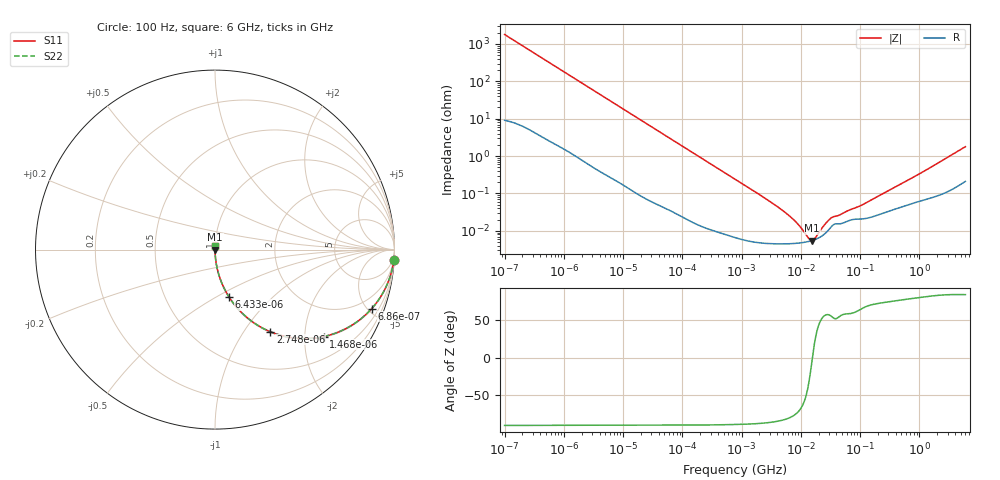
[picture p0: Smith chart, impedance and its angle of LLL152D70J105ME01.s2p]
!Murata Part Number: LLL152D70J105ME01
!These Parameters are Measured in Series Mode Connection
!Data Generated on Jan 08, 2026
!  o--ll--o
!Port1  Port2
!  o------o
!Operation Temp=25[degC], DC Bias Voltage=0[V]
!Freq. Start=100[Hz] Stop=6[GHz] 401[Steps]
# Hz S RI R 50
!Freq.(Hz) S11(Real) S11(Imag) S21(Real) S21(Imag) S12(Real) S12(Imag) S22(Real) S22(Imag)
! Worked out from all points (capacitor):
!   401 points, 100 Hz to 6 GHz, reference 50 ohm
!   read as one part in series: C = 885 nF near 109 Hz
!   lowest |Z| = 5.52 mohm at 15.56 MHz (marker M1)
!   series resonance near 15.7 MHz, so ESL is about 120 pH
!   S11 on the Smith chart (normalised r, x): 100 Hz: 1, -36; 686 Hz: 1.04, -5.29; 1.468 kHz: 1.02, -2.48; 2.748 kHz: 1.01, -1.33; 6.433 kHz: 1.01, -0.57; 6 GHz: 1.00, +0.04
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100  0.9966 -0.0555  0.00337 0.0555  0.00337 0.0555  0.9966 -0.0555
268  0.9774 -0.145  0.0226 0.145  0.0226 0.145  0.9774 -0.145
686  0.8727 -0.3292  0.1273 0.3292  0.1273 0.3292  0.8727 -0.3292
981  0.7721 -0.4153  0.2279 0.4153  0.2279 0.4153  0.7721 -0.4153
1468  0.605 -0.4845  0.395 0.4845  0.395 0.4845  0.605 -0.4845
2008  0.4523 -0.4935  0.5477 0.4935  0.5477 0.4935  0.4523 -0.4935
2748  0.308 -0.4574  0.692 0.4574  0.692 0.4574  0.308 -0.4574
4111  0.1675 -0.3692  0.8325 0.3692  0.8325 0.3692  0.1675 -0.3692
6433  0.0772 -0.2625  0.9228 0.2625  0.9228 0.2625  0.0772 -0.2625
15062  0.0158 -0.1203  0.9842 0.1203  0.9842 0.1203  0.0158 -0.1203
40335  0.00259 -0.0458  0.9974 0.0458  0.9974 0.0458  0.00259 -0.0458
774597  7.21e-05 -0.00244  0.9999 0.00244  0.9999 0.00244  7.21e-05 -0.00244
4643984  4.49e-05 -0.000374  1 0.000374  1 0.000374  4.49e-05 -0.000374
7266822  4.58e-05 -0.000206  1 0.000206  1 0.000206  4.58e-05 -0.000206
1.087309e7  4.87e-05 -9.15e-05  1 9.15e-05  1 9.15e-05  4.87e-05 -9.15e-05
1.189169e7  4.99e-05 -6.86e-05  1 6.86e-05  1 6.86e-05  4.99e-05 -6.86e-05
1.555665e7  5.52e-05 -2.2e-06  0.9999 2.2e-06  0.9999 2.2e-06  5.52e-05 -2.2e-06
2.035112e7  6.57e-05 6.44e-05  0.9999 -6.44e-05  0.9999 -6.44e-05  6.57e-05 6.44e-05
3.330331e7  0.000133 0.000184  0.9999 -0.000184  0.9999 -0.000184  0.000133 0.000184
1.020051e8  0.000208 0.000423  0.9998 -0.000423  0.9998 -0.000423  0.000208 0.000423
3.124326e8  0.000341 0.00118  0.9997 -0.00118  0.9997 -0.00118  0.000341 0.00118
6e9  0.00242 0.0177  0.9976 -0.0177  0.9976 -0.0177  0.00242 0.0177
